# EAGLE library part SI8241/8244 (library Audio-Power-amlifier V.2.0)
The Si824x isolated driver family combines two isolated drivers in a single package. The Si8241/44 are high-side/low-side drivers specifically targeted at high-power (>30 W) audio applications. Versions with peak output currents of 0.5 A (Si8241) and 4.0 A (Si8244) are available. All drivers operate with a maximum supply voltage of 24 V.
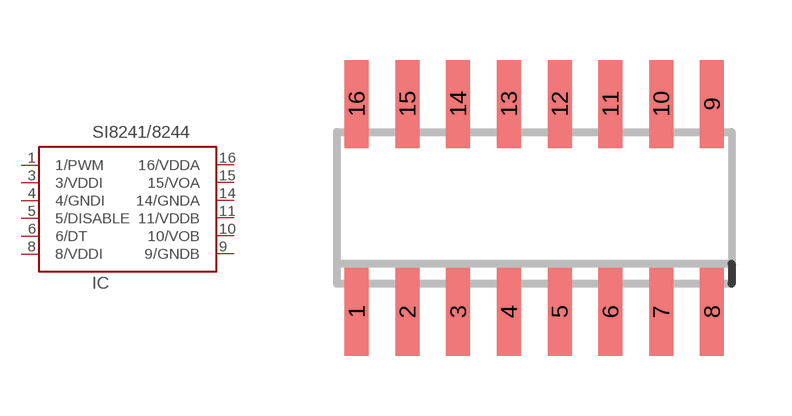
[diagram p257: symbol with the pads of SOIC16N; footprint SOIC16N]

Designator prefix IC

## SI8241/8244  [SOIC16N]
1  1/PWM  in
3  3/VDDI  in
4  4/GNDI  in
5  5/DISABLE  out
6  6/DT  in
8  8/VDDI  in
9  9/GNDB  pwr
10  10/VOB  out
11  11/VDDB  pwr
14  14/GNDA  pwr
15  15/VOA  out
16  16/VDDA  pwr

## Footprint SOIC16N (pad centres in mm)
SOIC16N SMALL OUTLINE INTEGRATED CIRCUIT NARROW
smd 0.6 x 2.2: 1 -4.445,-2.6; 2 -3.175,-2.6; 3 -1.905,-2.6; 4 -0.635,-2.6; 5 0.635,-2.6; 6 1.905,-2.6; 7 3.175,-2.6; 8 4.445,-2.6; 9 4.445,2.6; 10 3.175,2.6; 11 1.905,2.6; 12 0.635,2.6; 13 -0.635,2.6; 14 -1.905,2.6; 15 -3.175,2.6; 16 -4.445,2.6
